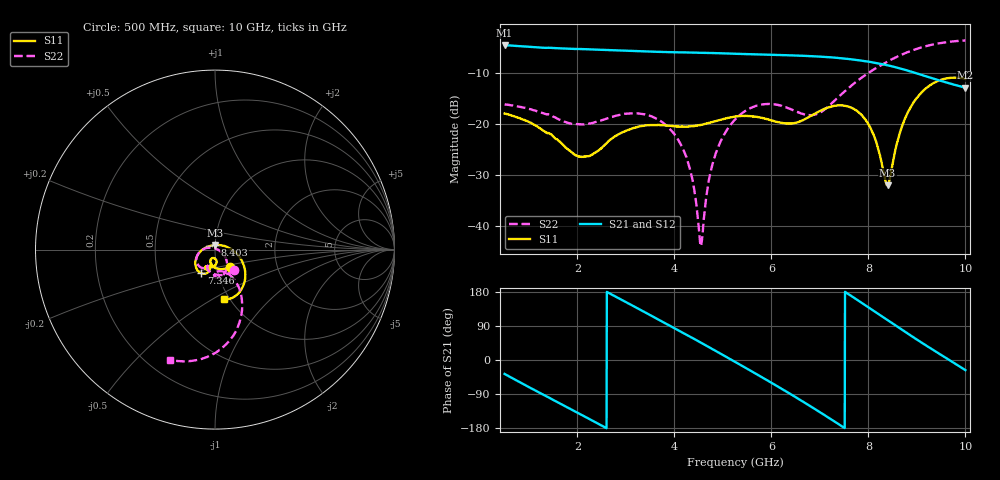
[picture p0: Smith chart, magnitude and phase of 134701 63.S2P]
!  2-Port S-parameters saved by WinCal
! VAR MeasName=S-Parameters (CALIBRATED_DATA) read from VNA (N5242A)
! VAR MeasDate=2013-7-3 16:41:42
! VAR NAME=134701 63
! VAR FILENAME=134701 63.S2P
! VAR DATE=2013-7-3 16:41:42
! VAR PHYS_PORTS=1,2
# Hz S MA R 50
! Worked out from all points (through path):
!   1601 points, 500 MHz to 10 GHz, reference 50 ohm
!   highest |S21| = -4.49 dB at 500 MHz (marker M1); lowest = -12.8 dB at 10 GHz (marker M2)
!   group delay of S21, straight-line fit = 207 ps
!   lowest |S11| = -32.0 dB at 8.397 GHz (marker M3), VSWR 1.05, Z = 49.9 + j2.51 ohm
!   |S11| at or under -10 dB: start of sweep to end of sweep
!   |S22| runs from -43.9 to -3.6 dB; largest |S21 - S12| = 0.002
!   S11 on the Smith chart (normalised r, x): 500 MHz: 1.16, -0.22; 7.346 GHz: 0.83, -0.23; 8.403 GHz: 1.00, +0.05; 10 GHz: 0.94, -0.56
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5e8  0.1273 -48.1  0.5966 -36.8  0.5969 -36.8  0.1567 -47.8
1.28375e9  0.0873 -101.4  0.5627 -90.5  0.5632 -90.6  0.1283 -99.7
2.085312e9  0.04779 -100.8  0.5455 -144.7  0.5454 -144.8  0.09952 -114.4
2.815625e9  0.07775 -84.8  0.5292 165.4  0.5293 165.3  0.1216 -121.9
3.670625e9  0.09823 -104.1  0.5128 107.0  0.5117 107.0  0.1106 -157.2
4.240625e9  0.09474 -107.0  0.5058 67.4  0.5052 67.4  0.04841 169.6
4.389062e9  0.0959 -105.9  0.5035 57.0  0.5039 57.0  0.02598 155.5
4.549375e9  0.09843 -105.1  0.5016 45.6  0.5019 45.6  0.006369 69.0
4.697812e9  0.1025 -104.6  0.4997 35.0  0.4998 35.0  0.02585 -13.6
4.804688e9  0.1057 -104.7  0.4986 27.3  0.4985 27.3  0.04367 -24.4
5.25e9  0.1187 -109.6  0.4908 -4.9  0.4912 -5.0  0.1111 -52.4
6.110938e9  0.1054 -118.0  0.4773 -68.3  0.4771 -68.3  0.1549 -88.6
6.835312e9  0.1219 -105.6  0.465 -124.5  0.4655 -124.5  0.1226 -79.1
7.345938e9  0.1523 -119.8  0.4477 -165.9  0.4483 -166.0  0.1784 -58.2
7.963438e9  0.1069 -160.0  0.413 142.3  0.4128 142.2  0.3094 -61.3
8.396875e9  0.02514 91.4  0.3782 105.1  0.3774 104.9  0.4112 -69.8
8.402812e9  0.0257 87.7  0.3775 104.6  0.3769 104.4  0.4127 -70.0
8.420625e9  0.0268 75.2  0.3758 102.9  0.3748 102.8  0.4171 -70.4
8.675938e9  0.09023 1.9  0.3494 81.2  0.3497 81.0  0.4787 -76.7
8.97875e9  0.1762 -26.7  0.3168 55.7  0.3169 55.5  0.5448 -85.2
9.45375e9  0.2676 -57.3  0.2695 17.1  0.2695 17.0  0.6202 -98.6
1e10  0.2791 -79.5  0.2283 -26.7  0.228 -26.9  0.6623 -112.1
